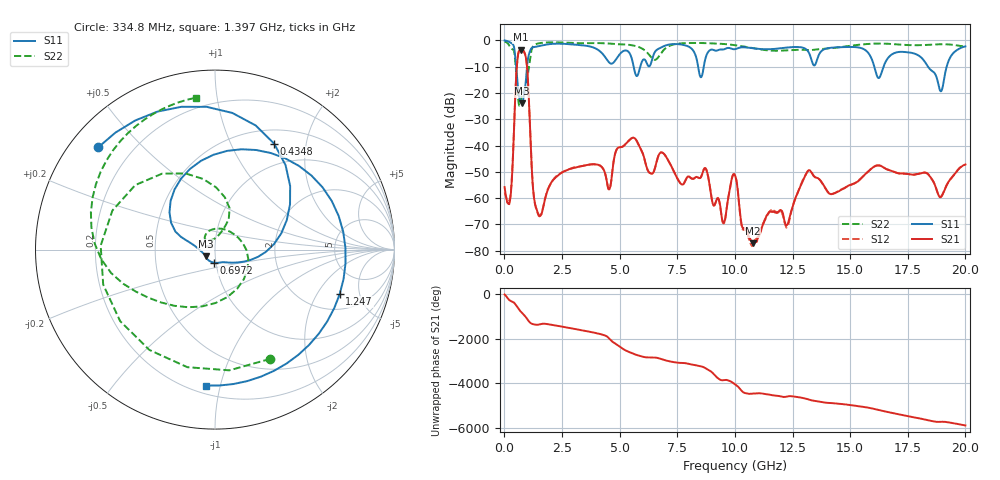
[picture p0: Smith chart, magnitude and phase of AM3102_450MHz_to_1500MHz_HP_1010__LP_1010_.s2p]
!Agilent Technologies,E8364B,MY43040894,A.07.50.67
!Agilent E8364B: A.07.50.67
!Date: Thursday, January 11, 2018 06:12:48
!Correction: S11(Full 2 Port(1,2))
!S21(Full 2 Port(1,2))
!S12(Full 2 Port(1,2))
!S22(Full 2 Port(1,2))
!S2P File: Measurements: S11, S21, S12, S22:
# Hz S  dB  R 50
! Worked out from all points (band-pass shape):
!   1601 points, 10 MHz to 20 GHz, reference 50 ohm
!   highest |S21| = -3.51 dB at 722.1 MHz (marker M1); lowest = -77.2 dB at 10.78 GHz (marker M2)
!   |S21| within 3 dB of the highest: 578 MHz to 931.6 MHz (353.6 MHz wide, 46.8 % of centre)
!   lowest |S11| = -23.9 dB at 759.6 MHz (marker M3), VSWR 1.14, Z = 44.9 - j3.35 ohm
!   |S11| at or under -10 dB: 513.5 MHz to 981.2 MHz (467.7 MHz wide, 62.6 % of centre); 16.05 GHz to 16.45 GHz (402.9 MHz wide, 2.48 % of centre); 18.37 GHz to 19.19 GHz (813.3 MHz wide, 4.33 % of centre)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
!   |S22| runs from -24.9 to -0.4 dB; largest |S21 - S12| = 0.00091
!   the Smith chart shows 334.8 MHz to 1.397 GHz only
!   S11 on the Smith chart (normalised r, x): 334.8 MHz: 0.08, +0.37; 434.8 MHz: 0.68, +1.48; 697.2 MHz: 0.97, -0.14; 1.247 GHz: 2.96, -3.21; 1.397 GHz: 0.25, -0.90
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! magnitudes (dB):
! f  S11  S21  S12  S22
! 10 MHz  -0.1  -55.8  -57.8  -0.4
! 334.8 MHz  -1.3  -51.4  -50.6  -3.3
! 434.8 MHz  -3.4  -29.6  -29.4  -4.9
! 697.2 MHz  -22.7  -3.5  -3.5  -24.1
! 722.1 MHz  -23.1  -3.5  -3.5  -23.1
! 759.6 MHz  -23.9  -3.6  -3.6  -20.7
! 984.5 MHz  -9.7  -10.3  -10.3  -15.2
! 1.247 GHz  -2.6  -56.8  -56.7  -2.3
! 1.397 GHz  -2.4  -64.2  -64.3  -1.4
! 3.346 GHz  -1.9  -47.9  -47.8  -1.1
! 4.545 GHz  -8.4  -56.7  -56.6  -1.2
! 4.895 GHz  -6.6  -41.2  -41.2  -1.5
! 5.745 GHz  -13.6  -38.3  -38.3  -2.3
! 6.682 GHz  -3.3  -43.9  -43.9  -6.4
! 8.731 GHz  -6.6  -48.7  -48.7  -1.1
! 9.505 GHz  -3.5  -69.3  -69.6  -1.4
! 10.01 GHz  -3.4  -51.3  -51.2  -1.9
! 10.78 GHz  -3.0  -77.2  -77.6  -3.0
! 13.34 GHz  -8.0  -50.5  -50.5  -3.7
! 16.68 GHz  -6.4  -49.3  -49.2  -1.3
! 18.94 GHz  -19.4  -59.6  -59.4  -1.5
! 20 GHz  -2.3  -47.2  -47.3  -2.4
